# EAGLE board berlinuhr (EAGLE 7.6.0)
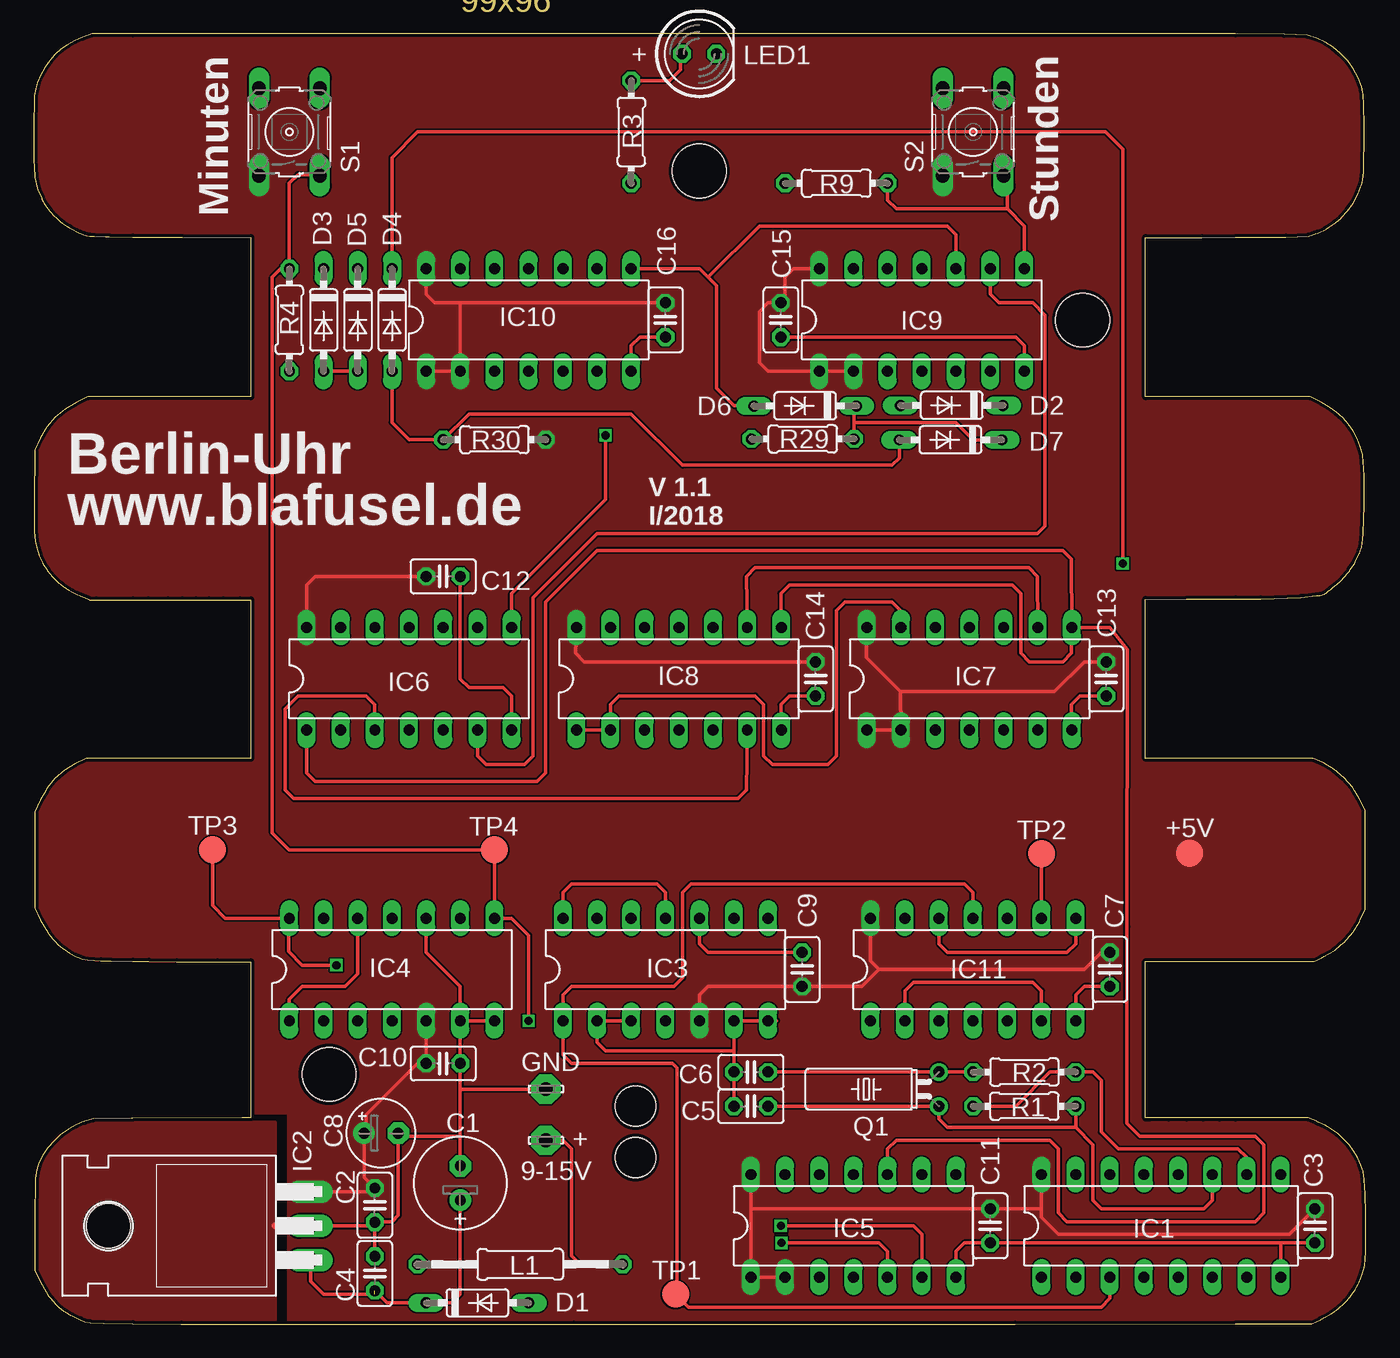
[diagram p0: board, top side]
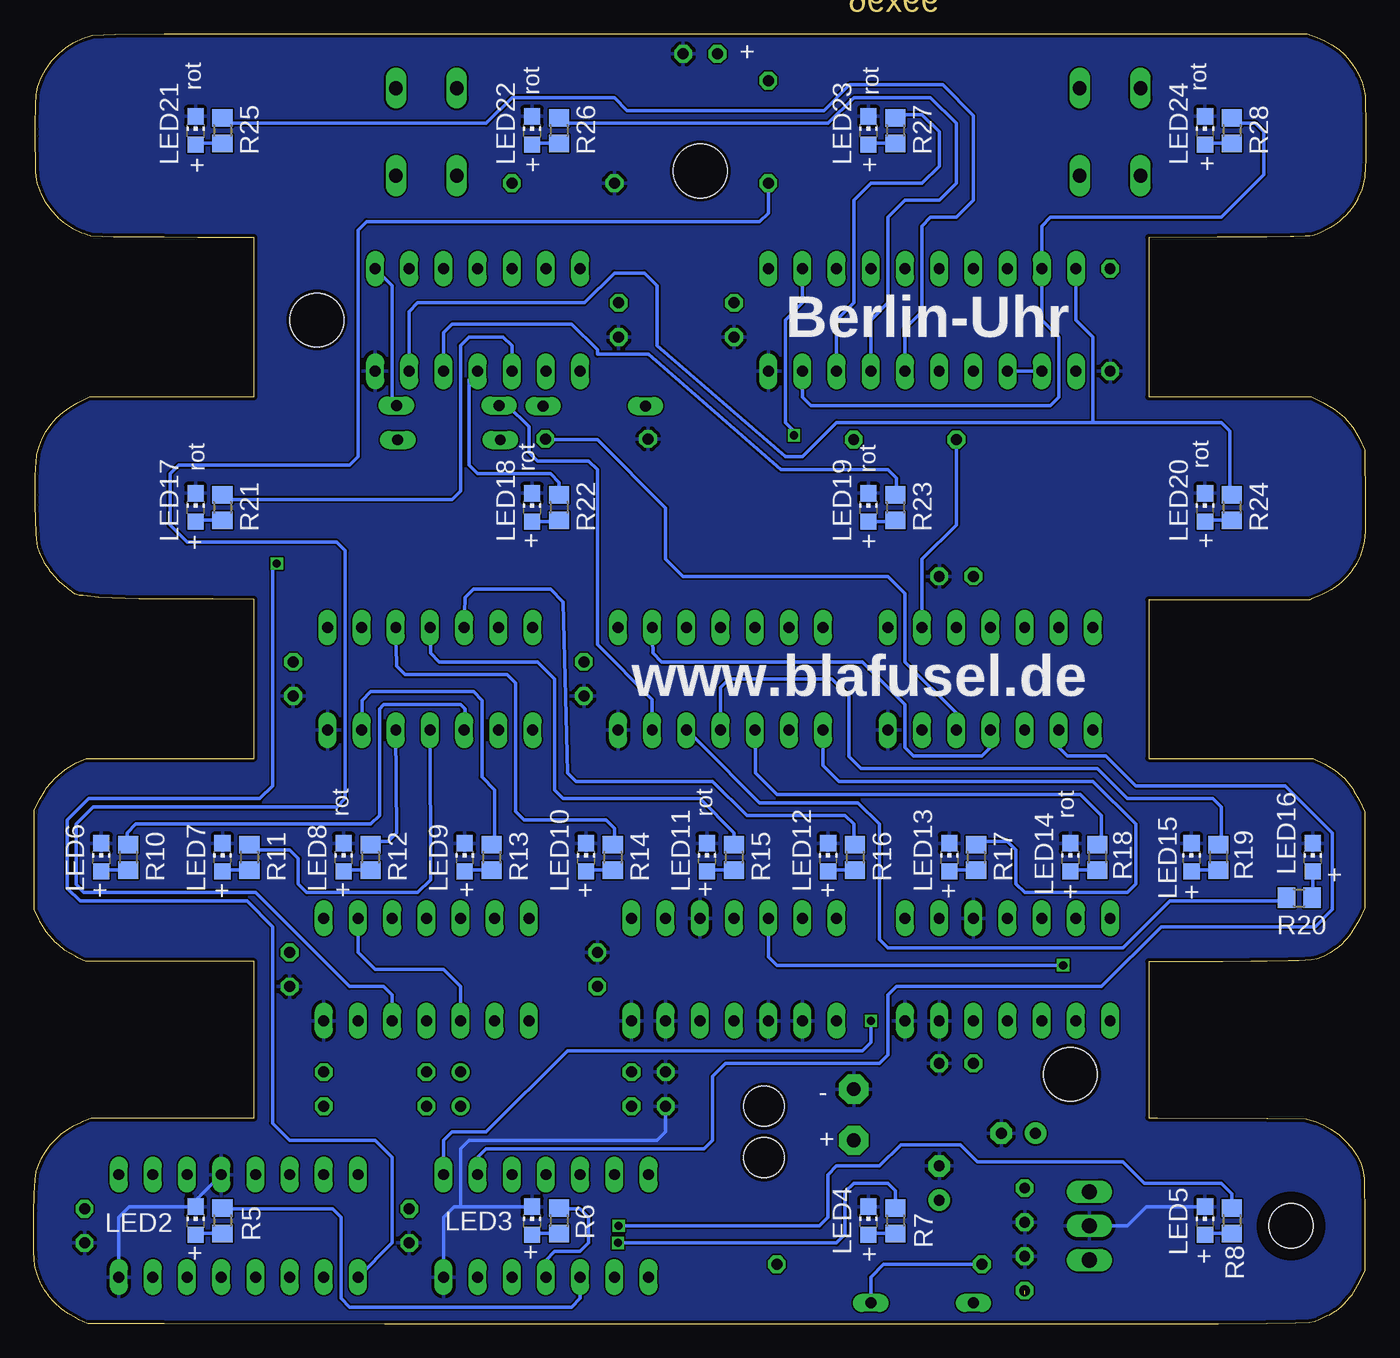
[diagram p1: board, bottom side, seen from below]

Size 98.98 x 95.89 mm. Coordinates in mm from the lower left corner, seen from the top.
Outline: 327 segments
Copper layers (1*16): Top 0.035mm / dielectric 1.5mm / Bottom 0.035mm
Design rules "dirt_cheap_dirty_boards.v1": minimum track width 5mil, minimum drill 12mil, track to track 5mil, track to pad 5mil, pad to pad 5mil, via to via 5mil, smd to smd 0mil, copper to edge 10mil, drill to drill 10mil, minimum pad ring 10mil, minimum via ring 6mil, stop-mask expansion 2mil, vias tented up to drill 25mil, thermal gap 10mil
Holes 3 mm at 44.72,16.2 44.72,12.39
Holes 4 mm at 49.45,85.69 21.94,18.57 77.94,74.62

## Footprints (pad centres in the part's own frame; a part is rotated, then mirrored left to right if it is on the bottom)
LSP10 = drill 1.016 pad 2.159 octagon: MP 0,0
TP20R = smd 2 x 2: TP 0,0
E2,5-7 = drill 0.813 pad 1.6: + -1.27,0 | drill 0.813 pad 1.6 octagon: - 1.27,0
C025-025X050 = drill 0.813 octagon: 1 -1.27,0; 2 1.27,0
E2,5-5 = drill 0.813 pad 1.6: + -1.27,0 | drill 0.813 pad 1.6 octagon: - 1.27,0
DO35-7 = drill 0.813 long: A 3.81,0; C -3.81,0
DIL16 = drill 0.813 long: 1 -8.89,-3.81; 2 -6.35,-3.81; 3 -3.81,-3.81; 4 -1.27,-3.81; 5 1.27,-3.81; 6 3.81,-3.81; 7 6.35,-3.81; 8 8.89,-3.81; 9 8.89,3.81; 10 6.35,3.81; 11 3.81,3.81; 12 1.27,3.81; 13 -1.27,3.81; 14 -3.81,3.81; 15 -6.35,3.81; 16 -8.89,3.81
TO220H = drill 1.118 long: 1 -2.54,-10.16; 2 0,-10.16; 3 2.54,-10.16 | hole 3.302: 0,4.826
DIL14 = drill 0.813 long: 1 -7.62,-3.81; 2 -5.08,-3.81; 3 -2.54,-3.81; 4 0,-3.81; 5 2.54,-3.81; 6 5.08,-3.81; 7 7.62,-3.81; 8 7.62,3.81; 9 5.08,3.81; 10 2.54,3.81; 11 0,3.81; 12 -2.54,3.81; 13 -5.08,3.81; 14 -7.62,3.81
0207/15 = drill 0.813 octagon: 1 -7.62,0; 2 7.62,0
LED5MM = drill 0.813 octagon: A -1.27,0; K 1.27,0
CHIP-LED0805 = smd 1.2 x 1.2: A 0,-1.05; C 0,1.05
TC38H = drill 0.813: 1 -1.27,0; 2 1.27,0
0204/7 = drill 0.813 octagon: 1 -3.81,0; 2 3.81,0
R0805 = smd 1.3 x 1.5: 1 -0.95,0; 2 0.95,0
B3F-10XX = drill 1.016 long: 1 -3.251,2.261; 2 3.251,2.261; 3 -3.251,-2.261; 4 3.251,-2.261

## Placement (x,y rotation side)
9-15V  LSP10  [LSP10]  38.05,13.66 0 top
+5V  TPTP20R  [TP20R]  85.9,35.01 0 top
C1  220µ/16V  [E2,5-7]  31.7,10.49 90 top
C2  100n  [C025-025X050]  25.35,8.85 270 top
C3  100n  [C025-025X050]  95.2,7.31 270 top
C4  100n  [C025-025X050]  25.35,3.77 90 top
C5  22p  [C025-025X050]  53.29,16.2 180 top
C6  22p  [C025-025X050]  53.29,18.74 180 top
C7  100n  [C025-025X050]  79.96,26.36 270 top
C8  10µ/6,3V  [E2,5-5]  25.81,14.2 0 top
C9  100n  [C025-025X050]  57.1,26.36 90 top
C10  100n  [C025-025X050]  30.43,19.38 0 top
C11  100n  [C025-025X050]  71.07,7.31 270 top
C12  100n  [C025-025X050]  30.43,55.57 0 top
C13  100n  [C025-025X050]  79.69,47.95 270 top
C14  100n  [C025-025X050]  58.1,47.95 270 top
C15  100n  [C025-025X050]  55.51,74.62 270 top
C16  100n  [C025-025X050]  46.94,74.62 270 top
D1  1N4148  [DO35-7]  32.97,1.6 0 top
D2  1N4148  [DO35-7]  68.21,68.27 180 top
D3  1N4148  [DO35-7]  21.54,74.62 270 top
D4  1N4148  [DO35-7]  26.62,74.62 270 top
D5  1N4148  [DO35-7]  24.08,74.62 270 top
D6  1N4148  [DO35-7]  57.32,68.24 180 top
D7  1N4148  [DO35-7]  68.12,65.71 180 top
GND  LSP10  [LSP10]  38.05,17.47 0 top
IC1  4060N  [DIL16]  83.77,7.31 0 top
IC2  7805T  [TO220H]  10.38,7.31 90 top
IC3  7490N  [DIL14]  46.94,26.36 0 top
IC4  74LS92N  [DIL14]  26.62,26.36 0 top
IC5  74164N  [DIL14]  60.91,7.31 0 top
IC6  7404N  [DIL14]  27.89,47.95 0 top
IC7  74164N  [DIL14]  69.53,47.95 0 top
IC8  74164N  [DIL14]  47.94,47.95 0 top
IC9  74164N  [DIL14]  65.99,74.62 0 top
IC10  74164N  [DIL14]  36.78,74.62 0 top
IC11  7474N  [DIL14]  69.8,26.36 0 top
L1  47µH/0,8A HBCC  [0207/15]  36.15,4.45 180 top
LED1  LED 5-3000 GE  [LED5MM]  49.45,94.39 0 top
LED2  ge, 20mA, 1V8, OF-SMD2012Y  [CHIP-LED0805]  86.95,7.69 0 bottom
LED3  [CHIP-LED0805]  61.95,7.69 0 bottom
LED4  [CHIP-LED0805]  36.95,7.69 0 bottom
LED5  [CHIP-LED0805]  11.95,7.69 0 bottom
LED6  ge, 20mA, 1V8, OF-SMD2012Y  [CHIP-LED0805]  93.95,34.69 0 bottom
LED7  [CHIP-LED0805]  84.95,34.69 0 bottom
LED8  rt, 20mA, 1V9, OF-SMD2012R  [CHIP-LED0805]  75.95,34.69 0 bottom
LED9  [CHIP-LED0805]  66.95,34.69 0 bottom
LED10  [CHIP-LED0805]  57.95,34.69 0 bottom
LED11  rt, 20mA, 1V9, OF-SMD2012R  [CHIP-LED0805]  48.95,34.69 0 bottom
LED12  [CHIP-LED0805]  39.95,34.69 0 bottom
LED13  [CHIP-LED0805]  30.95,34.69 0 bottom
LED14  rt, 20mA, 1V9, OF-SMD2012R  [CHIP-LED0805]  21.95,34.69 0 bottom
LED15  [CHIP-LED0805]  12.95,34.69 0 bottom
LED16  [CHIP-LED0805]  3.95,34.69 0 bottom
LED17  rt, 20mA, 1V9, OF-SMD2012R  [CHIP-LED0805]  86.95,60.69 0 bottom
LED18  [CHIP-LED0805]  61.95,60.69 0 bottom
LED19  [CHIP-LED0805]  36.95,60.69 0 bottom
LED20  [CHIP-LED0805]  11.95,60.69 0 bottom
LED21  rt, 20mA, 1V9, OF-SMD2012R  [CHIP-LED0805]  86.95,88.69 0 bottom
LED22  [CHIP-LED0805]  61.95,88.69 0 bottom
LED23  [CHIP-LED0805]  36.95,88.69 0 bottom
LED24  [CHIP-LED0805]  11.95,88.69 0 bottom
Q1  32,768  [TC38H]  67.26,17.47 90 top
R1  10M  [0204/7]  73.61,16.2 0 top
R2  220k  [0204/7]  73.61,18.74 180 top
R3  100  [0204/7]  44.4,88.59 270 top
R4  1k  [0204/7]  19,74.62 90 top
R5  150  [R0805]  84.95,7.69 270 bottom
R6  150  [R0805]  59.95,7.69 270 bottom
R7  150  [R0805]  34.95,7.69 270 bottom
R8  150  [R0805]  9.95,7.69 270 bottom
R9  1k  [0204/7]  59.64,84.78 0 top
R10  150  [R0805]  91.95,34.69 270 bottom
R11  150  [R0805]  82.95,34.69 270 bottom
R12  180  [R0805]  73.95,34.69 270 bottom
R13  150  [R0805]  64.95,34.69 270 bottom
R14  150  [R0805]  55.95,34.69 270 bottom
R15  180  [R0805]  46.95,34.69 270 bottom
R16  150  [R0805]  37.95,34.69 270 bottom
R17  150  [R0805]  28.95,34.69 270 bottom
R18  180  [R0805]  19.95,34.69 270 bottom
R19  150  [R0805]  10.95,34.69 270 bottom
R20  150  [R0805]  4.95,31.69 0 bottom
R21  180  [R0805]  84.95,60.69 270 bottom
R22  180  [R0805]  59.95,60.69 270 bottom
R23  180  [R0805]  34.95,60.69 270 bottom
R24  180  [R0805]  9.95,60.69 270 bottom
R25  180  [R0805]  84.95,88.69 270 bottom
R26  180  [R0805]  59.95,88.69 270 bottom
R27  180  [R0805]  34.95,88.69 270 bottom
R28  180  [R0805]  9.95,88.69 270 bottom
R29  1k  [0204/7]  57.15,65.78 0 top
R30  1k  [0204/7]  34.24,65.73 0 top
S1  Minuten  [B3F-10XX]  19,88.59 90 top
S2  Stunden  [B3F-10XX]  69.8,88.59 90 top
TP1  TPTP20R  [TP20R]  47.71,2.23 0 top
TP2  TPTP20R  [TP20R]  74.88,34.98 0 top
TP3  TPTP20R  [TP20R]  13.29,35.25 0 top
TP4  TPTP20R  [TP20R]  34.24,35.25 0 top

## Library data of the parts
9-15V GND = solpad
+5V TP1-TP4 = testpad
C1-C16 L1 R1-R30 = rcl
D1-D7 = diode
IC1 = 40xx
IC2 = linear
IC3-IC10 = 74xx-eu
IC11 = 74ttl-din
LED1-LED24 = led
Q1 = crystal; OC_FARNELL: unknown; OC_NEWARK: unknown
S1 S2 = switch-omron; MPN: B3F-1000; OC_FARNELL: 176432; OC_NEWARK: 36M3542

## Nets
+5V: +5V.TP C2.1 C3.1 C7.1 C8.+ C9.1 C10.1 C11.1 C12.1 C13.1 C14.1 C15.1 C16.1 IC1.16 IC2.3 IC3.5 IC4.5 IC5.1 IC5.2 IC5.14 IC6.14 IC7.1 IC7.2 IC7.14 IC8.14 IC9.1 IC9.2 IC9.14 IC10.1 IC10.2 IC10.14 IC11.14 R30.2 S1.1 S2.1
DIV12: D4.C IC1.1
GND: C1.- C2.2 C3.2 C4.2 C5.2 C6.2 C7.2 C8.- C9.2 C10.2 C11.2 C12.2 C13.2 C14.2 C15.2 C16.2 GND.MP IC1.8 IC1.12 IC2.2 IC3.2 IC3.3 IC3.6 IC3.7 IC3.10 IC4.6 IC4.7 IC4.10 IC5.7 IC6.7 IC7.7 IC8.7 IC9.7 IC10.7 IC11.7 LED1.K LED2.C LED3.C LED4.C LED5.C LED6.C LED7.C LED8.C LED9.C LED10.C LED11.C LED12.C LED13.C LED14.C LED15.C LED16.C LED17.C LED18.C LED19.C LED20.C LED21.C LED22.C LED23.C LED24.C R4.1 R9.1 R29.1
N$1: D1.A L1.2
N$2: C1.+ C4.1 D1.C IC2.1
N$3: LED1.A R3.1
N$4: C6.1 Q1.2 R2.2
N$5: C5.1 IC1.11 Q1.1 R1.2
N$6: IC1.10 R1.1 R2.1
N$7: IC11.5 R3.2
N$8: 9-15V.MP L1.1
N$9: IC1.3 IC3.1 IC11.11 TP1.TP
N$10: IC11.8 IC11.12
N$11: IC11.3 IC11.9 TP2.TP
N$12: IC11.2 IC11.6
N$13: IC3.11 IC3.14
N$14: LED2.A R5.2
N$15: IC3.12 IC4.14 TP3.TP
N$16: IC5.3 R5.1
N$17: LED3.A R6.2
N$18: IC4.8 IC5.8 R4.2 S1.3 TP4.TP
N$19: LED4.A R7.2
N$20: LED5.A R8.2
N$21: IC5.4 R6.1
N$22: IC5.5 R7.1
N$23: IC5.6 R8.1
N$24: IC4.1 IC4.12
N$25: IC5.9 IC6.2
N$26: D2.C IC9.8 R9.2 S2.3
N$27: IC6.6 IC9.9
N$28: IC5.10 IC6.1 IC7.8 IC8.8
N$29: IC7.13 IC8.1 IC8.2 R17.1
N$30: D2.A IC6.3 IC8.6
N$31: IC6.4 IC7.9 IC8.9
N$32: D3.A D4.A D5.A D7.A IC6.9 R30.1
N$33: LED6.A R10.2
N$34: IC7.3 R10.1
N$35: LED7.A R11.2
N$36: LED8.A R12.2
N$37: LED9.A R13.2
N$38: IC7.4 R11.1
N$39: IC7.5 R12.1
N$40: IC7.6 R13.1
N$41: LED10.A R14.2
N$42: IC7.10 R14.1
N$43: LED11.A R15.2
N$44: LED12.A R16.2
N$45: LED13.A R17.2
N$46: IC7.11 R15.1
N$47: IC7.12 R16.1
N$48: D6.C D7.C IC6.5 R29.2
N$49: LED14.A R18.2
N$50: IC8.3 R18.1
N$51: LED15.A R19.2
N$52: LED16.A R20.2
N$53: LED17.A R21.2
N$54: IC8.4 R19.1
N$55: IC8.5 R20.1
N$56: IC9.3 R21.1
N$57: LED18.A R22.2
N$58: LED19.A R23.2
N$59: LED20.A R24.2
N$60: IC9.4 R22.1
N$61: IC9.5 R23.1
N$62: D3.C IC9.6 R24.1
N$63: D6.A IC9.10 IC10.8
N$65: IC6.8 IC10.9
N$66: LED21.A R25.2
N$67: IC10.3 R25.1
N$68: LED22.A R26.2
N$69: LED23.A R27.2
N$70: LED24.A R28.2
N$71: IC10.4 R26.1
N$72: IC10.5 R27.1
N$73: D5.C IC10.6 R28.1

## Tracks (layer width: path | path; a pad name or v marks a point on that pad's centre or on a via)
+5V
  Top 0.254: 21.03,10.36 IC2.3 25.08,9.85 C2.1 24.54,10.93 C8.+ 24.72,14.38 24.72,15.57 28.53,19.38 C10.1 IC4.5 | 53.29,8.58 C11.1 74.88,8.58 | 53.29,8.58 IC5.14 | 74.88,8.58 IC1.16 | IC11.14 62.18,27 62.82,26.36 | IC3.5 49.48,24.46 50.12,25.09 C9.1 61.55,25.09 62.82,26.36 | IC7.14 61.86,49.54 64.4,47 | C12.1 20.91,55.57 20.27,54.94 IC6.14 | C16.1 31.7,75.89 | 31.7,75.89 29.8,75.89 29.16,76.53 IC10.14 | 53.29,8.58 IC5.1 IC5.2 | IC7.1 IC7.2 64.4,47 | IC10.1 IC10.2 31.7,75.89 | IC9.2 IC9.1 54.56,70.81 53.93,71.45 53.93,75.26 54.56,75.89 C15.1 55.83,76.21 55.83,77.8 56.47,78.43 58.05,78.43 | C7.1 79.33,27.63 78.06,26.36 62.82,26.36 | 64.4,47 75.83,47 78.06,49.22 C13.1 | C3.1 93.3,6.68 76.15,6.68 74.88,7.95 74.88,8.58 | C14.1 40.91,49.22 40.27,49.86 IC8.14
  pour Top (no thermals): -3.05,97.48 -3.32,15.69 18.95,15.69 18.95,-0.31 100.28,-0.31 100.28,97.48
DIV12  (via drill 0.6)
  Top 0.254: D4.C 26.62,86.69 28.53,88.59 79.64,88.59 80.91,87.32 v80.91,56.52
  Bottom 0.254: v80.91,56.52 81.23,56.21 81.23,40.01 82.18,39.06 94.88,39.06 96.47,37.47 96.47,32.39 95.52,31.44 83.14,31.44 81.23,29.54 81.23,14.93 79.96,13.66 73.61,13.66 72.34,12.39 72.34,6.04 IC1.1
GND
  Top 0.254: 31.51,11.63 C1.- 31.7,13.98 | GND.MP 31.7,17.47 | 31.7,17.47 31.7,13.98 | IC5.7 68.53,5.41 69.17,6.04 C11.2 92.66,6.04 | C3.2 92.66,6.04 | 92.66,6.04 IC1.8 | C7.2 78.06,25.09 77.42,24.46 IC11.7 | C9.2 50.12,27.63 49.48,28.27 IC3.10 | C13.2 77.74,46.68 77.1,46.05 IC7.7 | C14.2 56.15,46.68 55.51,46.05 IC8.7 | C12.2 31.7,47.95 32.34,47.32 34.88,47.32 35.51,46.68 IC6.7 | C16.2 45.04,73.35 44.4,72.72 IC10.7 | C5.2 C6.2 52.02,20.33 | 55.2,22.55 IC3.7 IC3.6 52.02,20.33 | IC4.6 IC4.7 | 52.02,20.33 42.5,20.33 41.86,20.96 IC3.2 IC3.3 | IC4.6 C10.2 31.7,17.47 | IC4.10 29.16,27.63 31.7,25.09 IC4.6 | C2.2 C4.2 | IC2.2 25.35,7.31 C2.2 | C2.2 25.4,7.63 26.62,7.63 27.08,8.09 C8.- 27.3,13.98 31.7,13.98 | C15.2 72.98,73.35 73.61,72.72 IC9.7
  Top 0.5: IC2.2 17.89,7.31
  Bottom 0.254: IC1.12 86.95,9.21 LED2.C 91.87,8.74 92.66,7.95 IC1.8 | LED3.C 67.26,8.74 | 67.26,8.74 67.74,8.74 68.53,7.95 IC5.7 | C5.2 52.02,14.3 52.66,13.66 66.63,13.66 67.26,13.03 67.26,8.74 | LED5.C 16.3,8.74 17.73,7.31 IC2.2
  pour Bottom: -2.59,97.48 105.36,97.48 105.36,-4.12 -2.59,-4.12
  pour Top (no thermals): -0.05,15.01 17.95,15.01 17.95,-0.31 -0.05,-0.31
N$1
  Bottom 0.254: L1.2 35.83,4.45 36.78,3.5 D1.A
N$2  (1 unrouted)
  Top 0.254: 25.35,2.23 21.54,2.23 20.59,3.18 20.59,4.72 IC2.1 | C4.1 26.26,1.6 D1.C 31.07,1.6 31.7,2.23 C1.+
N$3
  Top 0.254: R3.1 47.26,92.4 48.07,93.21 48.07,94.35 LED1.A
N$4
  Top 0.254: R2.2 Q1.2 C6.1
N$5
  Top 0.254: 77.42,14.61 68.21,14.61 67.9,14.61 67.26,15.25 Q1.1 C5.1 | IC1.11 87.58,9.22 86.95,8.58 79.33,8.58 78.69,9.22 78.69,13.34 77.42,14.61 | 77.42,14.61 R1.2
N$6
  Top 0.254: R1.1 72.98,16.2 75.52,18.74 R2.1 78.69,18.74 79.33,18.11 79.33,14.3 80.6,13.03 89.49,13.03 90.12,12.39 IC1.10
N$7
  Bottom 0.254: R3.2 44.4,82.56 45.04,81.92 74.25,81.92 74.88,81.29 74.88,64.46 75.52,63.83 88.22,63.83 88.85,63.19 88.85,59.38 87.58,58.11 76.47,58.11 75.83,57.48 75.83,39.06 76.42,38.43 94.57,38.43 95.84,37.16 95.84,32.66 95.25,32.08 82.5,32.08 75.52,25.09 72.98,25.09 72.34,24.46 IC11.5
N$8
  Top 0.254: L1.1 40.59,4.45 39.96,5.09 39.96,13.03 39.32,13.66 9-15V.MP
N$9
  Top 0.254: IC11.11 69.8,32.08 69.17,32.71 48.85,32.71 48.21,32.08 48.21,25.73 47.58,25.09 39.96,25.09 39.32,24.46 IC3.1 39.32,20.01 39.96,19.38 47.48,19.38 47.8,19.06 47.8,2.32 TP1.TP 48.66,1.28 79.33,1.28 79.96,1.91 IC1.3
N$10
  Top 0.254: IC11.12 67.26,28.27 67.9,27.63 76.79,27.63 77.42,28.27 IC11.8
N$11
  Top 0.254: TP2.TP IC11.9
  Bottom 0.254: IC11.3 67.26,25.09 68.53,26.36 73.61,26.36 74.88,27.63 IC11.9
N$12
  Top 0.254: IC11.6 74.88,24.77 74.25,25.41 65.36,25.41 64.72,24.77 IC11.2
N$13
  Top 0.254: IC3.11 46.94,32.08 46.31,32.71 39.96,32.71 39.32,32.08 IC3.14
N$14
  Bottom 0.254: R5.2 86.85,6.74 LED2.A
N$15  (via drill 0.6)
  Top 0.254: v22.49,26.68 19.96,26.68 18.95,27.69 18.95,30.12 IC4.14 14.24,30.17 13.29,31.12 TP3.TP
  Bottom 0.254: IC3.12 44.4,27.31 43.77,26.68 v22.49,26.68
N$16
  Bottom 0.254: 85.04,8.58 84.89,8.58 | IC5.3 58.37,1.91 59.01,1.28 75.52,1.28 76.15,1.91 76.15,7.95 76.79,8.58 84.89,8.58 | 84.89,8.58 R5.1
N$17
  Bottom 0.254: R6.2 61.85,6.74 LED3.A
N$18  (via drill 0.6)
  Top 0.254: v36.78,22.55 36.78,28.9 35.51,30.17 IC4.8 TP4.TP 19,35.25 17.73,36.52 17.73,77.8 18.37,78.43 R4.2 19,84.78 19.64,85.42 21.19,85.42 S1.3
  Bottom 0.254: v36.78,22.55 36.78,20.96 37.42,20.33 59.32,20.33 65.36,14.3 67.9,14.3 68.53,13.66 IC5.8
N$19
  Bottom 0.254: R7.2 36.85,6.74 LED4.A
N$20
  Bottom 0.254: R8.2 11.85,6.74 LED5.A
N$21
  Bottom 0.254: IC5.4 60.91,4.77 60.28,5.41 58.37,5.41 57.74,6.04 57.74,7.95 58.37,8.58 59.89,8.58 R6.1
N$22  (via drill 0.6)
  Top 0.254: v55.56,6.04 62.82,6.04 63.45,5.41 IC5.5
  Bottom 0.254: R7.1 34.95,9.93 35.51,10.49 38.05,10.49 38.69,9.85 38.69,6.68 39.32,6.04 v55.56,6.04
N$23  (via drill 0.6)
  Top 0.254: v55.51,7.31 65.36,7.31 65.99,6.68 IC5.6
  Bottom 0.254: R8.1 9.95,9.69 10.75,10.49 16.46,10.49 18.05,12.07 28.84,12.07 30.11,13.34 34.56,13.34 36.15,11.76 39.32,11.76 39.96,11.12 39.96,7.95 40.59,7.31 v55.51,7.31
N$24
  Top 0.254: IC4.1 19,24.14 19.95,25.09 23.13,25.09 24.08,26.04 IC4.12
N$25
  Bottom 0.254: IC6.2 22.81,42.87 22.18,42.24 19.32,42.24 17.1,40.01 5.98,40.01 2.49,36.52 2.49,30.81 3.76,29.54 15.19,29.54 19.64,25.09 34.88,25.09 35.51,24.46 35.51,20.01 36.15,19.38 47.58,19.38 48.53,18.42 48.53,13.66 49.16,13.03 65.36,13.03 65.99,12.39 IC5.9
N$26
  Top 0.254: R9.2 63.45,83.51 64.09,82.88 72.34,82.88 | 72.34,82.88 72.34,85.06 S2.3 | IC9.8 73.61,81.61 72.34,82.88
  Bottom 0.254: D2.C 72.34,68.27 72.34,77.16 IC9.8
N$27
  Top 0.254: IC6.6 32.97,42.24 33.61,41.6 36.46,41.6 37.1,42.24 37.1,53.98 41.86,58.75 74.56,58.75 75.13,59.32 75.13,74.97 74.25,75.89 71.71,75.89 71.07,76.53 IC9.9
N$28
  Top 0.254: IC7.8 77.1,49.86 76.47,49.22 73.98,49.22 73.34,49.86 73.34,54.3 72.71,54.94 56.15,54.94 55.51,54.3 IC8.8 | IC7.8 77.1,56.84 76.47,57.48 41.86,57.48 38.05,53.67 38.05,40.97 37.42,40.33 20.91,40.33 20.27,40.97 IC6.1 | IC5.10 63.45,13.03 64.09,13.66 75.52,13.66 76.15,13.03 76.15,8.26 76.79,7.63 90.76,7.63 91.39,8.26 91.39,13.34 90.76,13.98 82.18,13.98 81.23,14.93 81.23,29.54 81.28,50.13 79.96,51.76 IC7.8
N$29
  Top 0.254: IC8.1 IC8.2 42.86,46.05 43.5,46.68 53.61,46.68 54.24,46.05 54.24,42.24 54.88,41.6 59.01,41.6 59.64,42.24 59.64,53.03 60.28,53.67 63.77,53.67 64.4,53.03 IC7.13
  Bottom 0.254: IC8.1 40.32,41.51 39.15,40.33 20.27,40.33 17.1,37.16 17.1,32.71 17.73,32.08 25.35,32.08 25.99,32.71 25.99,35.25 26.62,35.89 28.71,35.89 R17.1
N$30
  Top 0.254: IC6.3 25.35,46.05 24.72,46.68 19.64,46.68 18.68,45.73 18.68,39.7 19.32,39.06 52.34,39.06 52.97,39.7 IC8.6
  Bottom 0.254: D2.A 63.77,68.27 62.18,66.68 62.18,64.78 61.55,64.14 57.74,64.14 57.1,63.51 57.1,50.49 53.02,46.41 IC8.6
N$31
  Top 0.254: IC8.9 52.97,55.57 53.61,56.21 73.93,56.21 74.56,55.57 IC7.9
  Bottom 0.254: IC8.9 52.97,49.86 52.34,49.22 37.42,49.22 34.24,46.05 34.24,42.87 33.61,42.24 28.53,42.24 27.89,42.87 IC6.4
N$32
  Top 0.254: D3.A D5.A | D4.A 26.62,67 27.89,65.73 R30.1 32.34,67.64 44.4,67.64 48.21,63.83 63.77,63.83 64.31,64.37 D7.A
  Bottom 0.254: D5.A D4.A | R30.1 30.43,59.38 32.97,56.84 IC6.9
N$33
  Bottom 0.254: R10.2 93.85,33.74 LED6.A
N$34
  Bottom 0.254: IC7.3 66.94,45.73 67.26,46.05 72.98,46.05 73.29,45.73 73.29,37.79 73.93,37.16 91.39,37.16 92.03,36.52 92.03,35.72 R10.1
N$35
  Bottom 0.254: R11.2 84.85,33.74 LED7.A
N$36
  Bottom 0.254: R12.2 75.85,33.74 LED8.A
N$37
  Bottom 0.254: R13.2 66.85,33.74 LED9.A
N$38
  Bottom 0.254: IC7.4 69.48,33.03 70.44,32.08 78.69,32.08 79.33,32.71 79.33,34.62 79.96,35.25 82.56,35.25 R11.1
N$39
  Bottom 0.254: IC7.5 72.02,36.52 72.66,35.89 73.71,35.89 R12.1
N$40
  Bottom 0.254: IC7.6 74.56,46.36 73.93,47 66.31,47 65.67,46.36 65.67,40.65 64.72,39.7 64.72,35.87 R13.1
N$41
  Bottom 0.254: R14.2 57.85,33.74 LED10.A
N$42
  Bottom 0.254: IC7.10 72.02,48.9 71.39,48.27 63.82,48.27 63.18,47.63 63.18,38.11 62.55,37.47 56.47,37.47 55.83,36.84 55.83,35.76 R14.1
N$43
  Bottom 0.254: R15.2 48.85,33.74 LED11.A
N$44
  Bottom 0.254: R16.2 39.85,33.74 LED12.A
N$45
  Bottom 0.254: R17.2 30.85,33.74 LED13.A
N$46
  Bottom 0.254: IC7.11 69.48,49.86 68.85,49.22 61.55,49.22 60.28,47.95 60.28,39.7 59.64,39.06 49.48,39.06 46.94,36.52 R15.1
N$47
  Bottom 0.254: IC7.12 66.94,53.98 66.31,54.62 60.59,54.62 59.64,53.67 59.32,40.97 58.69,40.33 48.53,40.33 45.99,37.79 38.69,37.79 38.05,37.16 38.05,35.74 R16.1
N$48
  Top 0.254: R29.2 60.96,67 | 60.96,67 60.96,68.06 D6.C | D7.C 69.82,65.71 68.53,67 60.96,67
  Bottom 0.254: R29.2 60.91,65.73 57.1,65.73 52.02,60.65 52.02,56.84 50.75,55.57 35.51,55.57 34.24,54.3 34.24,49.22 30.43,45.41 IC6.5
N$49
  Bottom 0.254: R18.2 21.85,33.74 LED14.A
N$50
  Bottom 0.254: R18.1 19.64,35.96 19.64,37.79 21.22,39.38 43.77,39.38 45.35,40.97 45.35,44.09 IC8.3
N$51
  Bottom 0.254: R19.2 12.85,33.74 LED15.A
N$52
  Bottom 0.254: LED16.A 3.95,31.74 R20.2
N$53
  Bottom 0.254: R21.2 86.85,59.74 LED17.A
N$54
  Bottom 0.254: IC8.4 47.94,47.32 47.31,47.95 39.69,47.95 38.42,46.68 38.42,42.19 37.51,41.28 19.95,41.28 17.73,39.06 11.38,39.06 10.75,38.43 10.75,35.85 R19.1
N$55
  Bottom 0.254: IC8.5 49.48,43.19 45.04,38.74 37.73,38.74 36.15,37.16 36.15,28.58 35.51,27.95 18.05,27.95 14.56,31.44 6.3,31.44 6.3,31.29 R20.1
N$56
  Bottom 0.254: IC9.3 63.45,72.72 64.09,73.35 66.63,73.35 67.26,72.72 67.26,61.92 67.9,61.29 84.6,61.29 R21.1
N$57
  Bottom 0.254: LED18.A 60.05,59.64 R22.2
N$58
  Bottom 0.254: LED19.A 35.05,59.64 R23.2
N$59
  Bottom 0.254: R24.2 11.85,59.74 LED20.A
N$60
  Bottom 0.254: R22.1 59.95,62.55 60.59,63.19 65.99,63.19 66.63,63.83 66.63,70.18 IC9.4
N$61
  Bottom 0.254: IC9.5 68.53,73.67 67.9,74.3 59.01,74.3 57.1,72.4 57.1,72.08 53.29,72.08 43.45,63.51 35.51,63.51 34.88,62.87 34.88,61.72 R23.1
N$62
  Bottom 0.254: IC9.6 71.07,75.26 70.44,75.89 58.05,75.89 55.83,78.11 53.61,78.11 52.66,77.16 52.66,72.72 43.13,64.46 41.86,64.46 39.32,67 20.27,67 | 20.27,67 10.75,67 10.11,66.37 10.11,61.8 R24.1 | D3.C 21.54,74.62 20.27,73.35 20.27,67
N$63
  Top 0.254: IC10.8 49.48,78.43 50.12,77.8 | 50.12,77.8 50.75,77.16 50.75,69.54 52.02,68.27 53.48,68.27 D6.A | IC9.10 68.53,80.97 67.9,81.61 53.93,81.61 50.12,77.8
N$65  (via drill 0.6)
  Top 0.254: IC6.8 35.51,54.3 42.5,61.29 v42.5,66.05
  Bottom 0.254: v42.5,66.05 42.5,66.37 43.13,67 43.13,74.62 41.86,75.89 IC10.9
N$66
  Bottom 0.254: R25.2 86.85,87.74 LED21.A
N$67
  Bottom 0.254: IC10.3 34.24,73.99 32.97,75.26 32.97,81.61 32.34,82.24 30.43,82.24 29.16,83.51 29.16,89.81 31.43,92.08 38.37,92.08 40.27,90.18 54.88,90.18 55.83,91.13 63.45,91.13 65.36,89.23 84.54,89.23 R25.1
N$68
  Bottom 0.254: R26.2 61.85,87.74 LED22.A
N$69
  Bottom 0.254: R27.2 36.85,87.74 LED23.A
N$70
  Bottom 0.254: R28.2 11.85,87.74 LED24.A
N$71
  Bottom 0.254: IC10.4 36.78,74.62 35.51,75.89 35.51,82.24 34.24,83.51 31.7,83.51 30.43,84.78 30.43,89.23 32.34,91.13 38.05,91.13 39.96,89.23 59.54,89.23 R26.1
N$72
  Bottom 0.254: IC10.5 39.32,74.62 38.05,75.89 38.05,83.51 36.78,84.78 32.97,84.78 31.7,86.05 31.7,88.59 32.97,89.86 34.73,89.86 R27.1
N$73
  Bottom 0.254: R28.1 9.54,89.23 8.21,89.23 7.57,88.59 7.57,85.42 10.75,82.24 23.45,82.24 24.08,81.61 D5.C 24.08,74.62 22.81,73.35 22.81,68.91 23.45,68.27 41.23,68.27 41.86,68.91 IC10.6

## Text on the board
Dimension: 99x96
tPlace: + | Minuten | Stunden | Berlin-Uhr | www.blafusel.de | V 1.1 / I/2018 | +
bPlace: rot | rot | rot | rot | Berlin-Uhr | rot | rot | rot | rot | www.blafusel.de | rot | rot | rot | - | +
bNames: + | + | + | + | + | + | + | + | + | + | + | + | + | + | + | + | + | + | + | + | + | + | + | +
tDocu: GND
